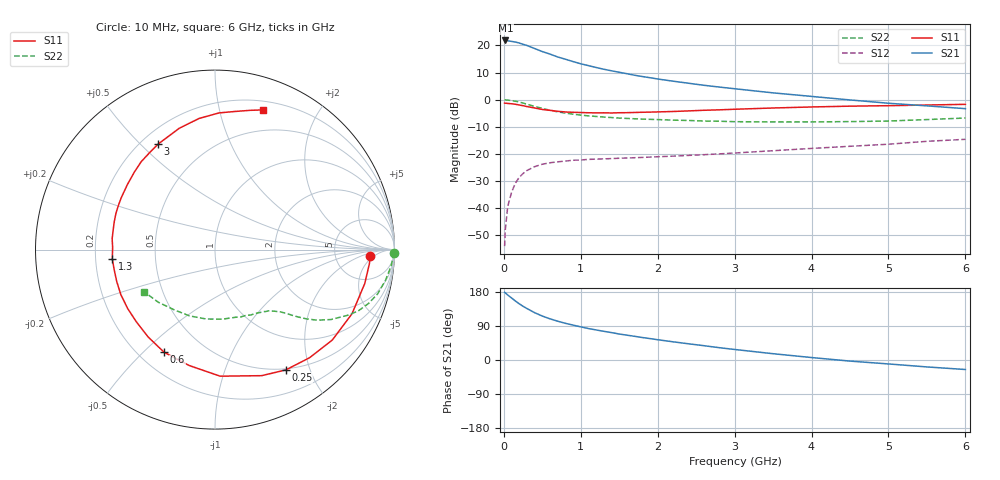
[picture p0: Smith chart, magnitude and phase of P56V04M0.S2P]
! SIEMENS Small Signal Semiconductors
! BFP183
! Si NPN RF Bipolar Junction Transistor in SOT143
! VCE = 6 V  IC = 4 mA
! Common Emitter S-Parameters:  March  1996
# GHz  S  MA  R  50
!  f  S11  S21  S12  S22
! GHz  MAG  ANG  MAG  ANG  MAG  ANG  MAG  ANG
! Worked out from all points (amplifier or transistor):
!   36 points, 10 MHz to 6 GHz, reference 50 ohm
!   highest |S21| = 21.9 dB at 20 MHz (marker M1)
!   |S21| within 3 dB of that: start of sweep to 402.9 MHz
!   unconditionally stable (mu >= 1): 1.756 GHz to 5.677 GHz
!   at 250 MHz: K = 0.18, MSG = 23.8 dB, |S12| = -27.2 dB
!   at 1.4 GHz: K = 0.85, MSG = 16.2 dB, |S12| = -21.7 dB
!   at 6 GHz: K = 0.94, MSG = 5.7 dB, |S12| = -14.6 dB
!   S11 on the Smith chart (normalised r, x): 10 MHz: 13, -4; 250 MHz: 0.48, -1.64; 600 MHz: 0.30, -0.58; 1.3 GHz: 0.27, -0.04; 3 GHz: 0.27, +0.57; 6 GHz: 0.28, +1.36
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0.01  0.8653 -2.5  12.32 178.4  0.002 87.0  0.9959 -1.0
0.02  0.8639 -5.2  12.38 177.0  0.0041 84.2  0.9931 -2.2
0.05  0.8555 -12.8  12.23 171.6  0.0107 85.6  0.9857 -5.3
0.15  0.8253 -37.6  11.58 155.7  0.029 70.0  0.9393 -15.2
0.2  0.8004 -48.8  11.11 148.4  0.0371 65.2  0.9066 -19.3
0.25  0.7779 -59.5  10.52 141.7  0.0437 59.1  0.869 -23.1
0.3  0.7489 -69.7  10.02 135.9  0.0496 55.2  0.8269 -26.2
0.4  0.7058 -87.7  8.801 124.9  0.0584 47.9  0.7544 -31.1
0.5  0.6615 -102.6  7.727 116.0  0.0648 41.9  0.6926 -34.6
0.6  0.6384 -116.4  6.94 108.6  0.0689 37.6  0.6406 -37.1
0.7  0.6128 -127.5  6.147 102.4  0.0717 34.3  0.5986 -38.9
0.8  0.5947 -137.6  5.587 96.8  0.0741 31.9  0.5668 -40.3
1  0.5815 -154.5  4.602 87.4  0.0775 28.7  0.5213 -42.5
1.1  0.5757 -161.9  4.256 83.0  0.0796 27.6  0.5042 -43.5
1.3  0.5744 -175.0  3.648 75.7  0.0814 26.1  0.4799 -45.7
1.7  0.5827 164.2  2.831 62.5  0.0854 25.5  0.4462 -50.6
2.2  0.6076 143.6  2.199 48.0  0.0913 26.2  0.4206 -57.8
3  0.6679 118.3  1.596 27.8  0.1043 27.9  0.3942 -73.0
3.5  0.7047 106.4  1.339 16.6  0.115 28.0  0.3897 -84.0
4.5  0.7619 88.3  0.992 -2.9  0.1387 25.9  0.3958 -111.1
5.5  0.7995 76.0  0.771 -18.3  0.1714 22.4  0.431 -137.1
6  0.8233 71.0  0.685 -25.1  0.1864 18.7  0.4604 -149.4
